FUNCTION "ROTAZIONE FLUSSAGGIO" : VOID
TITLE =ROTAZIONE FLUSSAGGIO
VERSION : 0.1

BEGIN
NETWORK
TITLE =ATTESA START ROTAZIONE
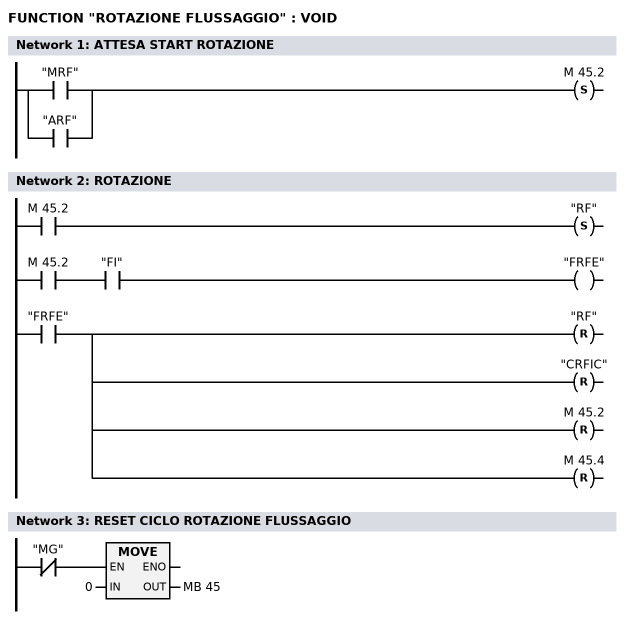
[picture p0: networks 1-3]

      U(    ;
      U     "MRF";
      O     ;
      U     "ARF";
      )     ;
//UN    "CRFIC"
      S     M     45.2;
// S     "CRFIC"
NETWORK
TITLE =ROTAZIONE

      U     M     45.2;
      S     "RF";
      U     M     45.2;
      U     "FI";
      =     "FRFE";
      U     "FRFE";
      R     "RF";
      R     "CRFIC";
      R     M     45.2;
      R     M     45.4;

NETWORK
TITLE =RESET CICLO ROTAZIONE FLUSSAGGIO

      UN    "MG";
      SPBN  FINE;
      L     0;
      T     MB    45;
FINE: NOP   0;
END_FUNCTION

